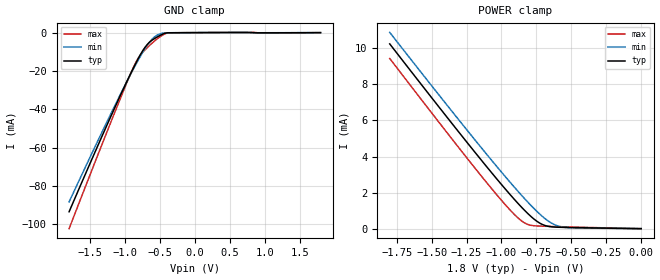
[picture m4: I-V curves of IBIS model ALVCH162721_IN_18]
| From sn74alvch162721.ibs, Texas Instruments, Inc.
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[Model]   ALVCH162721_IN_18
Model_type  Input
Vinl = 0.5775
Vinh = 1.2675
| variable   typ   min   max
C_comp   1.80pF   1.65pF   2.04pF
[Temperature Range]   40   100   -40
| Ambient temperature   25   85   -40
[Voltage range]   1.8   1.65   1.95
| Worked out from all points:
|   GND clamp passes 1 mA (typ) near -0.47 V on its own axis
|   POWER clamp passes 1 mA (typ) near -0.83 V on its own axis
[GND Clamp]
| ALVCH162721_IN_18
|   Voltage   I(typ)   I(min)   I(max)
-1.8V     -93.39mA   -88.25mA   -102.2mA
-1.235V   -46.33mA   -44.77mA   -49.66mA
-1V       -27.56mA   -27.45mA   -28.45mA
-875mV    -18.1mA    -18.66mA   -17.83mA
-795mV    -12.51mA   -13.33mA   -12.44mA
-700mV    -7.041mA   -7.586mA   -8.484mA
-615mV    -4.026mA   -3.532mA   -5.571mA
-540mV    -2.292mA   -1.342mA   -3.273mA
-445mV    -581uA     -184.1uA   -947.9uA
-375mV    -76.18uA   -61.83uA   -109.3uA
1.8V      25.63pA    20.14uA    -34.81uA
[POWER Clamp]
| ALVCH162721_IN_18
|   Voltage   I(typ)   I(min)   I(max)
-1.8V     10.24mA    10.88mA    9.436mA
-1.38V    6.082mA    6.753mA    5.225mA
-1.105V   3.426mA    4.114mA    2.544mA
-940mV    1.906mA    2.588mA    1.048mA
-885mV    1.428mA    2.099mA    619uA
-845mV    1.098mA    1.752mA    369.7uA
-795mV    718.3uA    1.336mA    196.1uA
-715mV    261.2uA    732.1uA    140.1uA
-645mV    105.9uA    322.9uA    123.4uA
-585mV    77.13uA    125.5uA    110.2uA
-480mV    58.79uA    41.84uA    88.08uA
-16.28fV  4.865pA    7.24pA     4.988pA
